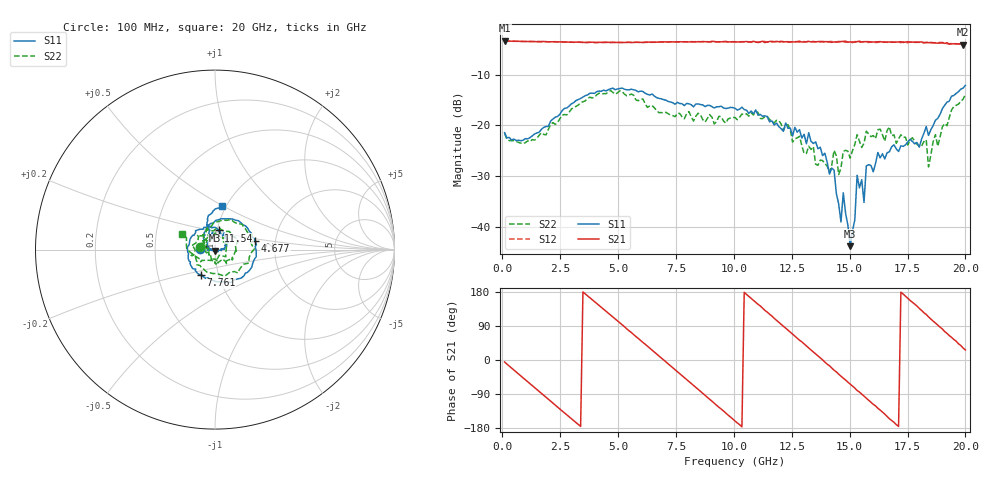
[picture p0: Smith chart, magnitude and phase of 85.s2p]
!Agilent Technologies,N5230C,MY49001569,A.09.33.09
!Agilent N5230C: A.09.33.09
!Date: Sunday, July 26, 2015 13:52:28
!Correction: S11(Full 2 Port(1,2))
!S21(Full 2 Port(1,2))
!S12(Full 2 Port(1,2))
!S22(Full 2 Port(1,2))
!S2P File: Measurements: S11, S21, S12, S22:
# Hz S  dB  R 50
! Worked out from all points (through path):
!   201 points, 100 MHz to 20 GHz, reference 50 ohm
!   highest |S21| = -3.31 dB at 100 MHz (marker M1); lowest = -4.1 dB at 19.9 GHz (marker M2)
!   group delay of S21, straight-line fit = 146 ps
!   lowest |S11| = -43.7 dB at 15.03 GHz (marker M3), VSWR 1.01, Z = 50 - j0.651 ohm
!   |S11| at or under -10 dB: start of sweep to end of sweep
!   |S22| runs from -29.6 to -13.1 dB; largest |S21 - S12| = 0.026
!   S11 on the Smith chart (normalised r, x): 100 MHz: 0.84, +0.01; 4.677 GHz: 1.57, +0.16; 7.761 GHz: 0.82, -0.24; 11.54 GHz: 1.02, +0.22; 20 GHz: 0.96, +0.50
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1e8  -21.42 177.3  -3.31 -5.3  -3.30 -5.2  -21.58 171.0
1.7915e9  -20.38 130.9  -3.51 -93.4  -3.53 -93.4  -21.76 143.4
3.483e9  -14.42 64.6  -3.66 179.6  -3.70 179.5  -15.35 74.4
4.677e9  -12.80 11.8  -3.67 118.3  -3.69 118.2  -13.14 21.3
5.672e9  -12.99 -30.9  -3.69 67.2  -3.66 66.9  -14.04 -22.6
6.7665e9  -14.68 -76.3  -3.61 10.5  -3.60 10.5  -17.50 -86.6
7.7615e9  -15.72 -118.9  -3.57 -41.5  -3.60 -41.6  -18.29 -146.4
8.856e9  -16.05 -156.4  -3.55 -98.6  -3.55 -98.8  -18.64 141.3
1.005e10  -16.62 147.0  -3.55 -161.1  -3.62 -161.3  -18.42 77.1
1.15425e10  -19.28 79.2  -3.50 121.0  -3.61 121.1  -18.79 -2.8
1.3433e10  -23.54 14.8  -3.49 21.2  -3.60 21.0  -24.17 -108.0
1.43285e10  -28.80 -8.2  -3.58 -26.9  -3.57 -26.7  -24.88 -171.0
1.4627e10  -38.97 -33.4  -3.51 -42.7  -3.58 -42.4  -28.32 168.6
1.47265e10  -33.22 -28.9  -3.47 -47.9  -3.54 -48.0  -25.09 164.3
1.5025e10  -43.72 -91.1  -3.57 -63.5  -3.59 -64.3  -26.44 173.1
1.53235e10  -29.80 179.3  -3.52 -80.4  -3.63 -79.9  -21.83 154.3
1.5622e10  -35.13 176.0  -3.53 -95.7  -3.57 -95.8  -23.49 131.1
1.57215e10  -27.97 -172.6  -3.52 -101.1  -3.52 -101.5  -21.12 136.2
1.67165e10  -25.17 132.3  -3.59 -155.1  -3.60 -154.1  -20.27 84.2
1.85075e10  -20.84 111.7  -3.69 108.2  -3.76 108.4  -25.84 -73.7
1.99005e10  -12.66 84.9  -4.14 31.8  -3.96 31.6  -14.83 156.7
2e10  -12.14 80.3  -3.99 26.4  -4.12 25.9  -13.93 154.6
